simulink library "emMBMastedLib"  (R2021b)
settings: Solver=VariableStepAuto  StartTime=0.0  StopTime=10.0  RelTol=1e-3
undefined symbols (not defined in the file or in its folder): A, Coils, Discretes, InputsReg, Read

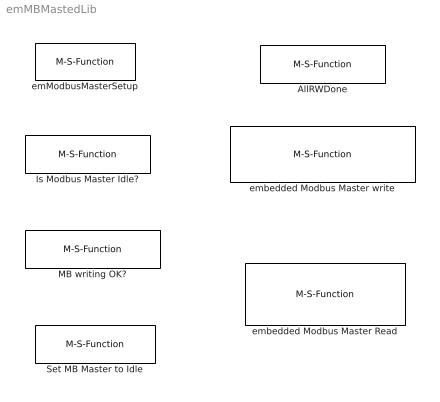
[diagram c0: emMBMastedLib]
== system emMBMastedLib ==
  AllRWDone : M-S-Function  FunctionName=AllWriteReadDone2  Parameters=c_sampleTime  mask(Are Modbus Master all Reading/Writing operaions done?){c_sampleTime=-1}
      mask prompts: c_sampleTime "Sample time in sec (-1 for inherited):"
      mask help: Judge whether embedded Modbus Master all reading/writing operations finish. Output Port "Yes" will be true when embedded Modbus master finish all reading/writing operations. After "Yes" is true, you must call "setMB2Idle" block in order to start new reading/writing operations for Modbus master
      mask init:
      | try
      |     set_param(gcs,'Lock',"off");
      |     set_param(gcbh,'MaskSelfModifiable',"on");
      | end
  Is Modbus Master Idle? : M-S-Function  Tag=isMB_Idle  FunctionName=isMB_Idle2  Parameters=c_sampleTime  mask(Is MB master in "Idle" State){c_sampleTime=-1}
      mask prompts: c_sampleTime "Sample time in sec (-1 for inherited):"
      mask help: Judge whether embedded Modbus Master is in "Idle" State. We do any "Modbus Master access to server" must be under condition : embedded Modbus Master is in "Idle" State. This block is for this purpose. Output Port "Yes" will be true when embedded Modbus master is in "Idle" State. However, when you call any "Reading or writing" block, Output Port "Yes" will be false.
      mask init:
      | try
      |     set_param(gcs,'Lock',"off");
      |     set_param(gcbh,'MaskSelfModifiable',"on");
      | end
  MB writing OK? : M-S-Function  FunctionName=isMB_WriteOK2  Parameters=c_writeNo,c_sampleTime  mask(judge whether Modbus master one sequence of writing to each modbus server success){c_writeNo=1, c_sampleTime=-1}
      mask prompts: c_writeNo "Command Seq No:"; c_sampleTime "Sample time in sec (-1 for inherited):"
      mask help: Judge whether embedded Modbus Master writing for specific sequence Number to each modbus server success. Output Port "Yes" is boolean scalar (if only one server for writing) or vector (if more servers for writing). Vector element is true means that related server writing operation success.
      mask init:
      | try
      |     set_param(gcs,'Lock',"off");
      |     set_param(gcbh,'MaskSelfModifiable',"on");
      | end
  Set MB Master to Idle : M-S-Function  Tag=setMB2Idle  FunctionName=setMB2Idle2  mask(Set embedded Modbus Master to idle state){}
      mask help: Judge whether embedded Modbus Master is in "Idle" State. We do any "Modbus Master access to server" must be under condition : embedded Modbus Master is in "Idle" State. This block is for this purpose. Output Port "Yes" will be true when embedded Modbus master is in "Idle" State. However, when you camm any "Reading or writing" block, Output Port "Yes" will be false.
      mask init:
      | try
      |     set_param(gcs,'Lock',"off");
      |     set_param(gcbh,'MaskSelfModifiable',"on");
      | end
  emModbusMasterSetup : M-S-Function  Tag=emModbusMasterSetup  FunctionName=emModbusMasterSetup2  Parameters=c_uartNo, c_baudrate,c_forceLongerSpace,c_writeServerID,c_writeCMD1Type,c_writeCMD2Type,c_writeCMD3Type,c_writeCMD4Type,c_writeCMD5Type,c_writeCMD6Type,c_writeCMD7Type,c_writeCMD8Type,c_writeCMD9Type,c_writeCMD10Type,c_writeCMD11Type,c_writeCMD12Type,c_writeCMD13Type,c_writeCMD14Type,c_writeCMD15Type,c_writeRegMAXQTY,c_readCMD1Type,c_readCMD2Type,c_readCMD3Type,c_readCMD4Type,c_readCMD5Type,c_read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  mask(embedded Modbus Master setup){c_uartNo=4, c_baudrate=9600, c_forceLongerSpace=on, c_writeServerID=[2  4 7 ], c_writeCMD1Type=Mask-write-holding, c_writeCMD2Type=Single-Write-coil, c_writeCMD3Type=Multiple-Write-coils, c_writeCMD4Type=Single-Write-holding, c_writeCMD5Type=Single-Write-holding, c_writeCMD6Type=Single-Write-holding, c_writeCMD7Type=Single-Write-holding, c_writeCMD8Type=Single-Write-holding, c_writeCMD9Type=Single-Write-holding, c_writeCMD10Type=Single-Write-holding, c_writeCMD11Type=Single-Write-holding, c_writeCMD12Type=Single-Write-holding, c_writeCMD13Type=Single-Write-holding, c_writeCMD14Type=Single-Write-holding, c_writeCMD15Type=Single-Write-holding, c_writeRegMAXQTY=[2 1 45], c_readCMD1Type=Read-InputsReg, c_readCMD2Type=Read-Discretes, c_readCMD3Type=Read-Coils, c_readCMD4Type=Read-Discretes, c_readCMD5Type=Read-InputsReg, c_readCMD6Type=Read-InputsReg, c_readCMD7Type=Read-InputsReg, c_readCMD8Type=Read-InputsReg, c_readCMD9Type=Read-InputsReg, c_readCMD10Type=Read-InputsReg, c_readCMD11Type=Read-InputsReg, c_readCMD12Type=Read-InputsReg, c_readCMD13Type=Read-InputsReg, c_readCMD14Type=Read-InputsReg, c_readCMD15Type=Read-InputsReg, c_readCMD16Type=Read-InputsReg, c_readRegMAXQTY=[30 7 200 300 5 6 7 8 9 10 11 12 13 14 15], c_MaxTry=10, c_Timeout=800, c_Name_method=By phycical port name and bit number, c_PortName=A, c_BitNo=7, c_txEnable485="LATAbits.LATA7", c_TxEnable485Polarity=on}
      mask prompts: c_uartNo "UART No:"; c_baudrate "Baud Rate:"; c_forceLongerSpace "Force longer space"; c_writeServerID "Servers Max Qty each writing action"; c_writeCMD1Type "The 1st Write command type:"; c_writeCMD2Type "The 2nd Write command type:"; c_writeCMD3Type "The 3rd Write command type:"; c_writeCMD4Type "The 4th Write command type:"; c_writeCMD5Type "The 5th Write command type:"; c_writeCMD6Type "The 6th Write command type:"; c_writeCMD7Type "The 7th Write command type:"; c_writeCMD8Type "The 8th Write command type:"; c_writeCMD9Type "The 9th Write command type:"; c_writeCMD10Type "The 10th Write command type:"; c_writeCMD11Type "The 11th Write command type:"; c_writeCMD12Type "The 12th Write command type:"; c_writeCMD13Type "The 13th Write command type:"; c_writeCMD14Type "The 14th Write command type:"; c_writeCMD15Type "The 15th Write command type:"; c_writeRegMAXQTY "Register Max QTY:"; c_readCMD1Type "The 1st Read command type:"; c_readCMD2Type "The 2nd Read command type:"; c_readCMD3Type "The 3rd Read command type:"; c_readCMD4Type "The 4th Read command type:"; c_readCMD5Type "The 5th Read command type:"; c_readCMD6Type "The 6th Read command type:"; c_readCMD7Type "The 7th Read command type:"; c_readCMD8Type "The 8th Read command type:"; c_readCMD9Type "The 9th Read command type:"; c_readCMD10Type "The 10th Read command type:"; c_readCMD11Type "The 11th Read command type:"; c_readCMD12Type "The 12th Read command type:"; c_readCMD13Type "The 13th Read command type:"; c_readCMD14Type "The 14th Read command type:"; c_readCMD15Type "The 15th Read command type:"; c_readCMD16Type "The 16th Read command type:"; c_readRegMAXQTY "Register Max QTY:"; c_MaxTry "Try Times when error occurs"; c_Timeout "Modbus Master Timeout in ms"; c_Name_method "How to specify Tx Enable Port:"; c_PortName "Port Name:"; c_BitNo "Port Bit number::"; c_txEnable485 "Tx Enable C Var/Func for RS485"; c_TxEnable485Polarity "Tx Enable control Polarity for RS485 is High"
      mask help: Set up embedded Modbus Client (Master) Parameters. If you create Modbus Master in your firmware, you must have this block. All mosbus master operations are in Sequence. Only when Modbus master is in "idle" state, it can run Sequence. The maximum sequence QTY for writing operation is 15. In any writing operation sequence, you can write as manay as 20 Modbus Servers which has the same registers address and writing values. The maximum sequence QTY for reading operation is 16. In any reading operation sequence, you can read only one Modbus Server. If at the same time, Both Writing operation and Re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
      mask init:
      | try
      |     set_param(gcs,'Lock',"off");
      |     set_param(gcbh,'MaskSelfModifiable',"on");
      | end
  embedded Modbus Master Read : M-S-Function  Tag=ModbusMasterReading  FunctionName=emModbusMasterRead2  Parameters=c_SeverID,c_readNo,c_readType,c_dataType,c_dataQTY,c_endian  mask(embedded Modbus Master reading registers){c_SeverID=1, c_readNo=1, c_readType=Read-InputsReg, c_dataType=Unsigned 16 bits int, c_dataQTY=1, c_endian=Big-endian}
      mask prompts: c_SeverID "Server ID:"; c_readNo "Command Seq No:"; c_readType "Read Operation type:"; c_dataType "Data Output Type"; c_dataQTY "Data Output Vector Length"; c_endian "Word-Endian when multiple Words"
      mask help: This block will execute Modbus Master reading operation in one sequence number. It is only executing its reading when Input port "En" is true. "En" generally connects output port of block "isMB_Idle" in order to make sure reading only when Modbus master is in "Idle" state. Output port "Done" is logical scalar. True means reading operation has finished (it may success or may fail). Output port "Success" is logical scalar. True means reading operation success. Output port "Data" is data result for reading. It could be scalar or vector. It is decided by parameter "Data Output Vector Length" Data 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
      mask init:
      | try
      |     set_param(gcs,'Lock',"off");
      |     set_param(gcbh,'MaskSelfModifiable',"on");
      | end
  embedded Modbus Master write : M-S-Function  Tag=ModbusMasterWriting  FunctionName=emModbusMasterWrite2  Parameters=c_SeverID,c_writeNo,c_writeType,c_endian  mask(embedded Modbus Master writing register(s)){c_SeverID=1, c_writeNo=1, c_writeType=Single-Write-holding, c_endian=Big-endian}
      mask prompts: c_SeverID "Server IDs:"; c_writeNo "Command Seq No:"; c_writeType "Write Operation type:"; c_endian "Word-Endian when multiple Words"
      mask help: This block will execute Modbus Master writing operation in one sequence number. It is only executing its writing when Input port "En" is true. "En" generally connects output port of block "isMB_Idle" in order to make sure writing only when Modbus master is in "Idle" state. Input port "Data" is Data source for writing. It could be scalar or vector. Data type could be "uint8/int8/uint16/int16/uint32/int32/single". It cannot be "uint64/int64/double". If writing to coil registers, Data type should be "boolean". Output port "Done" is logical scalar. True means wrting operation has finished (it may 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
      mask init:
      | try
      |     set_param(gcs,'Lock',"off");
      |     set_param(gcbh,'MaskSelfModifiable',"on");
      | end
